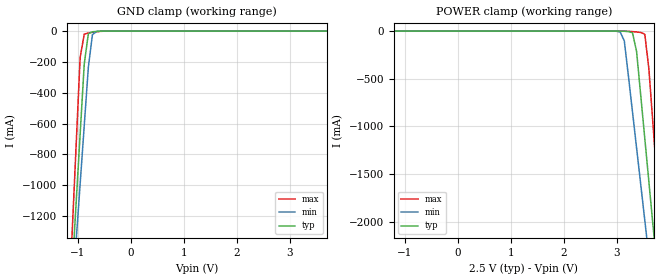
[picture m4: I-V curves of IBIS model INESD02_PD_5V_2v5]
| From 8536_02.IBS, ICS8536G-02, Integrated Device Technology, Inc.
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[Model] INESD02_PD_5V_2v5
Model_type   Input
Polarity   Non-Inverting
Vinl = .87V
Vinh = 1.62V
|   typ   min   max
C_comp   2pF   1.5pF   2.5pF
|   typ   min   max
[Voltage range]   2.5V   2.375V   2.625V
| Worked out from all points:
|   GND clamp passes 1 mA (typ) near -0.59 V on its own axis
[GND_clamp]
|Voltage   I(typ)   I(min)   I(max)
-2.191V   -7.973A    -7.07A     -9.504A
-1.108V   -1.581A    -1.751A    -1.338A
-1.031V   -1.125A    -1.371A    -755.2mA
-953.6mV  -669.5mA   -992.5mA   -172.1mA
-876.3mV  -213.9mA   -613.7mA   -19.96mA
-799mV    -17.31mA   -235.3mA   -12.11mA
-721.6mV  -4.455mA   -23.01mA   -7.724mA
-644.3mV  -1.863mA   -2.522mA   -4.06mA
5V        97.41uA    121.8uA    75.48uA
[POWER_clamp]
|Voltage   I(typ)   I(min)   I(max)
-2.5V     97.41uA    118.8uA    77.37uA
2.835V    -9.233uA   -44.7uA    -3.208uA
3.067V    -617.5uA   -9.489mA   -116.3uA
3.144V    -1.863mA   -101.8mA   -642.8uA
3.299V    -17.31mA   -847.2mA   -5.362mA
3.376V    -213.9mA   -1.226A    -9.326mA
3.531V    -1.125A    -1.985A    -32.65mA
3.608V    -1.581A    -2.364A    -395.6mA
3.686V    -2.038A    -2.744A    -978.8mA
3.763V    -2.494A    -3.124A    -1.562A
3.84V     -2.95A     -3.503A    -2.145A
4.845V    -8.886A    -8.445A    -9.728A
